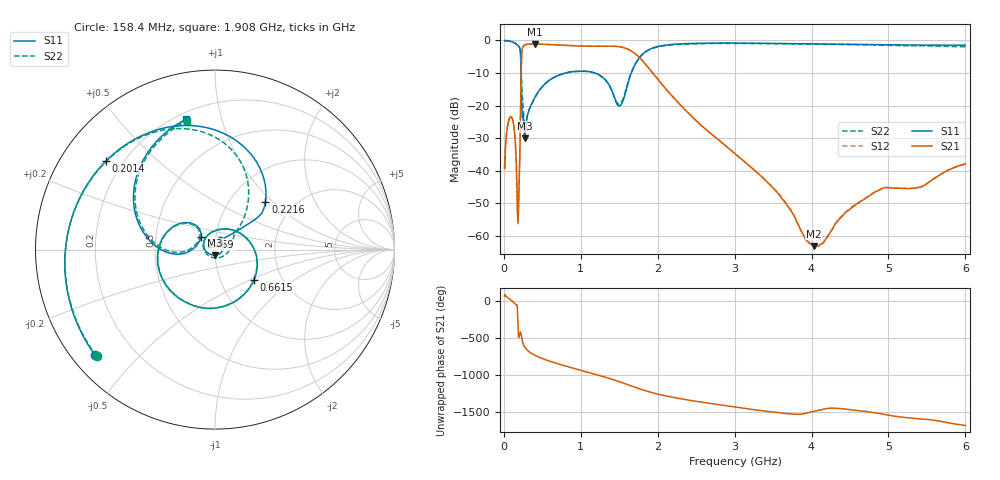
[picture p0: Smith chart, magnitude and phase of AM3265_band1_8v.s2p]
!Agilent Technologies,E8364B,MY43040894,A.07.50.67
!Agilent E8364B: A.07.50.67
!Date: Friday, May 09, 2025 07:17:45
!Correction: S11(Full 2 Port(1,2))
!S21(Full 2 Port(1,2))
!S12(Full 2 Port(1,2))
!S22(Full 2 Port(1,2))
!S2P File: Measurements: S11, S21, S12, S22:Log Frequency Sweep
# Hz S  dB  R 50
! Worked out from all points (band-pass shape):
!   3201 points, 10 MHz to 6 GHz, reference 50 ohm
!   highest |S21| = -1.11 dB at 401.3 MHz (marker M1); lowest = -63.1 dB at 4.031 GHz (marker M2)
!   |S21| within 3 dB of the highest: 233.4 MHz to 1.709 GHz (1.476 GHz wide, 152 % of centre)
!   lowest |S11| = -30.0 dB at 271.2 MHz (marker M3), VSWR 1.07, Z = 50.1 - j3.17 ohm
!   |S11| at or under -10 dB: 222.7 MHz to 799.8 MHz (577 MHz wide, 113 % of centre); 1.185 GHz to 1.656 GHz (470.6 MHz wide, 33.1 % of centre)
!   |S22| runs from -26.7 to -0.1 dB; largest |S21 - S12| = 0.0041
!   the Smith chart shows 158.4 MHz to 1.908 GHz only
!   S11 on the Smith chart (normalised r, x): 158.4 MHz: 0.07, -0.37; 201.4 MHz: 0.14, +0.35; 221.6 MHz: 1.45, +0.91; 661.5 MHz: 1.44, -0.52; 1.469 GHz: 0.85, +0.12; 1.908 GHz: 0.24, +0.78
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1e7  -0.07 -7.3  -38.94 67.7  -39.01 76.0  -0.07 -7.2
2.908064e7  -0.06 -20.9  -30.19 70.5  -30.16 70.1  -0.07 -20.9
8.439949e7  -0.24 -63.0  -23.49 25.6  -23.50 25.9  -0.28 -63.2
1.584215e8  -1.02 -138.8  -35.59 -43.3  -35.39 -42.4  -1.04 -138.0
1.818519e8  -1.51 -175.0  -55.56 92.6  -56.20 144.2  -1.50 -172.8
2.0137e8  -2.13 140.9  -42.32 -108.7  -42.30 -109.0  -2.07 146.5
2.216496e8  -8.25 43.4  -13.59 -73.0  -13.53 -72.9  -6.25 71.2
2.44949e8  -22.74 70.1  -2.21 161.8  -2.18 161.8  -18.27 32.1
2.712392e8  -29.99 -86.9  -1.40 100.4  -1.35 100.3  -26.46 -84.4
4.013416e8  -17.55 59.7  -1.11 -11.7  -1.08 -11.8  -17.71 61.9
6.615417e8  -11.22 -37.6  -1.35 -115.4  -1.32 -115.4  -11.24 -37.8
7.123273e8  -10.69 -52.2  -1.41 -131.8  -1.38 -131.8  -10.70 -52.6
1.141743e9  -9.71 -167.7  -1.78 101.3  -1.76 101.3  -9.77 -168.6
1.468784e9  -19.48 137.5  -1.84 -0.2  -1.81 -0.2  -19.07 139.6
1.908484e9  -2.57 102.4  -9.21 -155.9  -9.18 -155.9  -2.67 102.1
2.067357e9  -1.56 62.8  -13.80 163.3  -13.78 163.3  -1.68 63.2
2.450248e9  -0.92 -10.2  -23.49 88.5  -23.47 88.7  -1.05 -9.5
2.962692e9  -0.79 -89.2  -33.94 7.8  -33.91 7.8  -0.90 -89.4
3.504394e9  -0.90 -164.6  -45.39 -67.1  -45.30 -66.1  -1.00 -166.4
4.030742e9  -1.06 126.3  -63.07 -56.3  -62.89 -58.4  -1.17 123.9
5.002045e9  -1.35 4.3  -45.20 -108.8  -45.21 -109.4  -1.53 4.8
6e9  -1.45 -115.2  -37.91 112.2  -38.02 113.6  -1.96 -111.0
